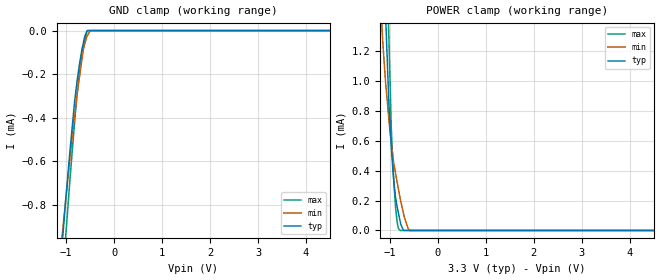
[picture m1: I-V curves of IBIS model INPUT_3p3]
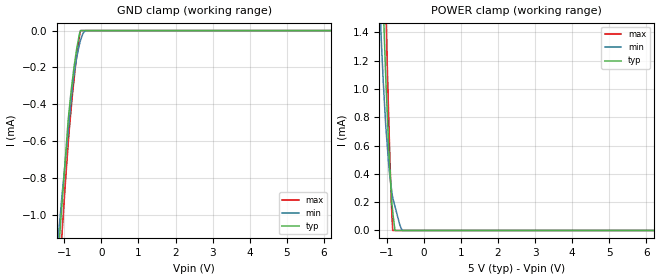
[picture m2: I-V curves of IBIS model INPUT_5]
|Texas Instruments Incorporated
|16-Bit, Ultralow Glitch Voltage Output DAC
| Marketing part#   Digital Voltage Range   Package-type   #pins
| DAC8550IBDGKR   2.7V to 5.5V   MSOP   8
| DAC8550IBDGKRG4   2.7V to 5.5V   MSOP   8
| DAC8550IBDGKT   2.7V to 5.5V   MSOP   8
| DAC8550IBDGKTG4   2.7V to 5.5V   MSOP   8
| DAC8550IDGKR   2.7V to 5.5V   MSOP   8
| DAC8550IDGKRG4   2.7V to 5.5V   MSOP   8
| DAC8550IDGKT   2.7V to 5.5V   MSOP   8
| DAC8550IDGKTG4   2.7V to 5.5V   MSOP   8
[IBIS Ver]   3.2
[File name]   dac8550.ibs
|SIMDE Ver   V2.0 - 201002 - RHL4 - Build 372
[Date]   07/08/2010
[File Rev]   1.2
[Source]
| Texas Instruments Incorporated.
| Analog eLab Design Center, HPA
| 12500 TI Blvd
| Dallas, TX -75243
| e-Mail: elab_scm_ibis@list.ti.com
| Model generated from simulations in TISPICE
[Notes]   Revision_History:
|   Rev 1.0: 06/11/2010
|   - Initial version of the model
|   - Initial Model generated from simulations in TIspiceD
|   - Model names with a trailing _3p3 contains the model for
|   3.3V [2.7V and 3.6V]. Model names with trailing _5 contains
|   the model for 5V [4.5V and 5.5V] operation.
|   Rev 1.1: 06/25/2010
|   - Model generated from simulations in TISPICE
|   - Model matched to SPICE simulation
|   - Updated the ibis file with data sheet title and package
|   details
|   - While calculating R_pkg, L_pkg and C_pkg ignored values
|   corresponding to power and ground pins
|   - C_comp although listed in numerical order of value are
|   obtained from varying PVT conditions. For PVT conditions
|   for each specific value refer the buffer description under
|   respective [Model]. IBIS model user is responsible for using
|   appropriate C_comp to simulate for Signal Integrity.
|   Rev 1.2: 07/08/2010
|   - Added package details beside [Package]
|   - Removed C_comp (ON state) and C_comp (OFF state) lines
[Disclaimer]
| This model is designed as an aid for customers of Texas Instruments.
| TI and its licensors and suppliers make no warranties, either expressed
| or implied, with respect to this  model, including the warranties of
| merchantability or fitness for a particular purpose. The model is
| provided solely on an "as is" basis. The entire risk as to its quality
| and performance is with the customer.
[Copyright]
| (C) Copyright 2010 Texas Instruments Incorporated. All rights reserved.
|   DAC8550
[Component]   DAC8550
[Manufacturer]  TI
[Package]   | 8 MSOP - DGK package
| variable   typ   min   max
R_pkg   0.048445   0.03118   0.06571
L_pkg   1.537895nH   1.35098nH   1.72481nH
C_pkg   0.40488pF   0.37893pF   0.43083pF
|-------------------------PIN------------------------------------------------
[Pin]  signal_name model_name   R_pin   L_pin   C_pin
1   VDD   POWER   0.03466   1.49519nH   0.40511pF
2   VREF   NC   0.03187   1.35098nH   0.43083pF
3   VFB   NC   0.03118   1.36336nH   0.42413pF
4   VOUT   NC   0.03481   1.50355nH   0.40491pF
5   _SYNC   INPUT   0.06571   1.72481nH   0.37893pF
6   SCLK   INPUT   0.0589   1.58493nH   0.39579pF
7   Din   INPUT   0.05834   1.57275nH   0.39607pF
8   GND   GND   0.03528   1.51429nH   0.40424pF
|   Model Selectors
[Model Selector]  INPUT
INPUT_3p3  3V digital input
INPUT_5   5V digital input
| Models and submodels in the file (2): INPUT_3p3 (Input), INPUT_5 (Input)
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|NOTES   Model INPUT split into two Models INPUT_3p3 and INPUT_5
|   to accomodate vast voltage range of 2.7V - 5.5V
|   INPUT_3p3 operates in voltage range of 3 - 3.3 - 3.6
|   INPUT_5 operates in voltage range of 4.5 - 5 - 5.5
|   The max pin frequency for Model INPUT is 20MHz for 3v range
|   and 30.3MHz for 5v range.Also the voltage range and frequency
|   is referenced with datasheet.
|   Input INPUT 3V Model
[Model] INPUT_3p3
Model_type Input
| Signals   _SYNC(5), SCLK(6), Din(7)
Vinl = 0.6
Vinh = 2.1
|   typ   min   max
|   (nom PVT)   (Fast PVT)   (slow PVT)
C_comp   5.041e-13   4.621e-13   5.122e-13
| Where   nom PVT is  Nominal Process, 3.3V, 25C
|   Fast PVT is Strong Process, 3.6V, -40C
|   Slow PVT is Weak Process, 3.0V, 105C
[Voltage Range]   3.3   3   3.6
[Temperature Range]   25   105   -40
[Power Clamp Reference]   3.3   3   3.6
[GND Clamp Reference]   0   0   0
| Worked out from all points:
|   GND clamp passes 1 mA (typ) near -1.09 V on its own axis
|   POWER clamp passes 1 mA (typ) near -1.04 V on its own axis
[GND Clamp]
|   Voltage   I(typ)   I(min)   I(max)
-3.3V     -7.871mA   -6.18mA    -10.49mA
-1.136V   -1.137mA   -1.06mA    -1.344mA
-1.043V   -869.2uA   -851.3uA   -1.043mA
-1.016V   -796uA     -793uA     -965.4uA
-927.6mV  -570.2uA   -602.2uA   -704.9uA
-825mV    -329.3uA   -390.9uA   -425.6uA
-772.2mV  -232.4uA   -297.8uA   -290.7uA
-697.2mV  -121.4uA   -173.8uA   -154.5uA
-645mV    -59.96uA   -92.42uA   -82.6uA
-554.4mV  0A         -22.62uA   0A
-466.8mV  0A         0A         0A
6.6V      0A         0A         0A
[POWER Clamp]
|   Voltage   I(typ)   I(min)   I(max)
-3.3V     30.52mA    23.75mA    38.67mA
-1.165V   2.169mA    1.36mA     3.176mA
-1.086V   1.411mA    976.9uA    2.1mA
-1.057V   1.164mA    874.8uA    1.729mA
-1.02V    842uA      742uA      1.278mA
-970.8mV  563uA      589.3uA    689.2uA
-927.6mV  368.1uA    470.2uA    384.5uA
-884.4mV  229.3uA    388.3uA    168.5uA
-848.4mV  158.1uA    322.8uA    56.46uA
-783mV    57.27uA    210.3uA    0A
-574.8mV  0A         0A         0A
6.6V      0A         0A         0A
|   Input INPUT 5V Model
[Model] INPUT_5
Model_type Input
| Signals   _SYNC(5), SCLK(6), Din(7)
Vinl = 0.8
Vinh = 2.4
|   typ   min   max
|   (nom PVT)   (Fast PVT)   (slow PVT)
C_comp   4.372e-13   4.306e-13   5.038e-13
| Where   nom PVT is  Nominal Process, 5.0V, 25C
|   Fast PVT is Strong Process, 5.5V, -40C
|   Slow PVT is Weak Process, 4.5V, 105C
[Voltage Range]   5   4.5   5.5
[Temperature Range]   25   105   -40
[Power Clamp Reference]   5   4.5   5.5
[GND Clamp Reference]   0   0   0
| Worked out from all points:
|   GND clamp passes 1 mA (typ) near -1.08 V on its own axis
|   POWER clamp passes 1 mA (typ) near -1.02 V on its own axis
[GND Clamp]
|   Voltage   I(typ)   I(min)   I(max)
-5V       -13.27mA   -10.27mA   -17.9mA
-1.172V   -1.238mA   -1.141mA   -1.465mA
-1.073V   -968.7uA   -917.7uA   -1.136mA
-1.062V   -940.2uA   -894uA     -1.104mA
-895mV    -484.4uA   -542.9uA   -613uA
-815mV    -326.2uA   -375.2uA   -422uA
-761mV    -235.4uA   -268.3uA   -309.3uA
-666.5mV  -99.96uA   -146.2uA   -140.7uA
-595mV    -21.4uA    -77.85uA   -38uA
-558.5mV  0A         -49.69uA   0A
-430mV    0A         0A         0A
10V       0A         0A         0A
[POWER Clamp]
|   Voltage   I(typ)   I(min)   I(max)
-5V       53.94mA    42.83mA    67.6mA
-1.177V   2.294mA    1.521mA    3.356mA
-1.15V    2.04mA     1.354mA    3.001mA
-1.099V   1.609mA    1.064mA    2.383mA
-1.062V   1.332mA    893.3uA    1.95mA
-1.025V   1.056mA    727.3uA    1.563mA
-979.5mV  776.3uA    571uA      1.086mA
-880.5mV  265.8uA    306.1uA    204.6uA
-837.5mV  124.5uA    228.3uA    0A
-780mV    0A         170.4uA    0A
-572.5mV  0A         0A         0A
10V       0A         0A         0A
